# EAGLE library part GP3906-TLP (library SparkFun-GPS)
GP3906-TLP PoT GPS Module The GP3906-TLP is a POT (Patch on Top) GPS module which is special designed for ultra low power consumption purpose environment. It is a GPS receiver providing a solution that high position and speed accuracy performances as well as high sensitivity and tracking capabilities in urban conditions. The GPS chipsets inside the module are designed by MediaTek Inc., which is the world's leading digital media solution provider and largest fab-less IC company in Taiwan. The module can support up to 66 channels. The GPS solution enables small form factor devices. They deliver major advancements in GPS performances, accuracy, integration, computing power and flexibility. They are designed to simplify the embedded system integration process. Features: Based on MediaTek Single Chip Architecture (MT3339). ARM7 based application processor High sensitivity: -165dBm tracking L1 frequency, C/A code Channels: 66 acquisition, 22 simultaneous tracking Low power consumption: 26mA @ acquisition, 20mA @ tracking Cold/Warm/Hot start time: Maximum update rate up to 10Hz GPS data interface: TTL level serial port Support NMEA 0183 standard V3.01 and backward compliance Support SBAS – WAAS, EGNOS, GAGAN and MSAS Dimension：16mm x 16mm x 6.7mm RoHS compliant Advanced software features AlwaysLocate TM advanced location awareness technology EPO TM orbit prediction Supports logger function (LOCUS) SparkFun Products SparkFun GPS Logger Shield
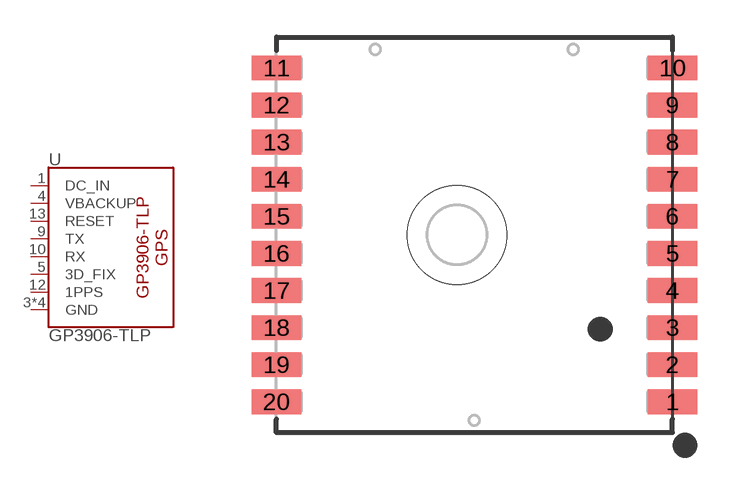
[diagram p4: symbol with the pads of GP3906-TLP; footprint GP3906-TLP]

Designator prefix U

## GP3906-TLP (PROD_ID: GPS-13174)  [GP3906-TLP]
1  DC_IN
3  GND
4  VBACKUP
5  3D_FIX
8  GND
9  TX
10  RX
11  GND
12  1PPS
13  RESET
20  GND

## Footprint GP3906-TLP (pad centres in mm)
GP3906-TLP PoT GPS Module The GP3906-TLP is a POT (Patch on Top) GPS module which is special designed for ultra low power consumption purpose environment. It is a GPS receiver providing a solution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
smd 2 x 1: 1 8,-6.75; 2 8,-5.25; 3 8,-3.75; 4 8,-2.25; 5 8,-0.75; 6 8,0.75; 7 8,2.25; 8 8,3.75; 9 8,5.25; 10 8,6.75; 11 -8,6.75; 12 -8,5.25; 13 -8,3.75; 14 -8,2.25; 15 -8,0.75; 16 -8,-0.75; 17 -8,-2.25; 18 -8,-3.75; 19 -8,-5.25; 20 -8,-6.75
hole 4 at -0.7,0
